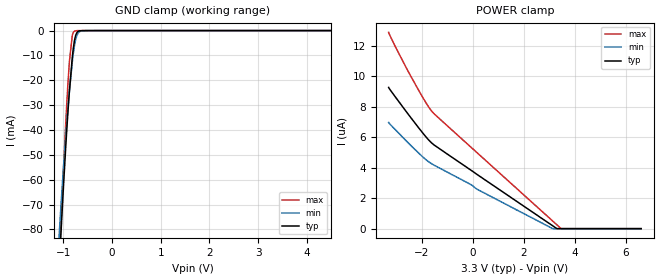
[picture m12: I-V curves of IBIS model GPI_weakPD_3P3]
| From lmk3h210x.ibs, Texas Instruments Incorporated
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[Model]   GPI_weakPD_3P3
Model_type   Input
Vinl = 0.99
Vinh = 2.31
|   typ   min   max
C_comp   0.55pF   0.44pF   0.66pF
[Voltage Range]   3.3   3.135   3.465
[Temperature Range]   45   125   -40
[Power Clamp Reference]   3.3   3.135   3.465
[GND Clamp Reference]   0   0   0
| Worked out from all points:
|   GND clamp passes 1 mA (typ) near -0.73 V on its own axis
[GND Clamp]
|   Voltage   I(typ)   I(min)   I(max)
-3.3V     -1.045A    -940.6mA   -1.157A
-1.142V   -118.3mA   -101.5mA   -119.5mA
-1.073V   -91.24mA   -78.45mA   -88.62mA
-1.043V   -79.98mA   -69.1mA    -75.68mA
-943.8mV  -44.99mA   -41.05mA   -35.22mA
-904.2mV  -32.74mA   -31.27mA   -21.28mA
-874.5mV  -24.48mA   -24.49mA   -12.51mA
-815.1mV  -10.84mA   -12.72mA   -2.002mA
-765.6mV  -3.561mA   -5.597mA   -216.9uA
-696.3mV  -357uA     -1.066mA   -24.74uA
-557.7mV  -13.06uA   -40.11uA   -14.63uA
6.6V      0A         0A         0A
[POWER Clamp]
|   Voltage   I(typ)   I(min)   I(max)
-3.3V     9.274uA    6.971uA    12.89uA
-3.023V   8.617uA    6.471uA    11.9uA
-2.419V   7.265uA    5.446uA    9.973uA
-1.835V   6.023uA    4.526uA    8.262uA
-1.567V   5.561uA    4.216uA    7.629uA
-102.3mV  3.874uA    2.919uA    5.394uA
214.5mV   3.504uA    2.547uA    4.915uA
3.125V    196.7nA    4.766nA    512.3nA
3.293V    4.788nA    0A         257.7nA
3.462V    0A         0A         3.096nA
6.6V      0A         0A         0A
